(* Logix 5000 AddOnInstructionDefinition export TeNod4TBlocBackupRestore; software revision 28.00 *)

ADD_ON_INSTRUCTION TeNod4TBlocBackupRestore   (* revision 1.1, vendor Scaime *)
VAR_IN_OUT
   Datas : TeNod4TDatas; {required}
END_VAR
VAR_INPUT
   Backup : BOOL; {visible}
   Restore : BOOL; {visible}
END_VAR
VAR_OUTPUT
   InProgress : BOOL; {visible}
   Done : BOOL; {visible}
   Error : BOOL; {visible}
END_VAR
VAR
   IntBackup : BOOL; {access None}
   IntRestore1 : BOOL; {access None}
   IntRestore2 : BOOL; {access None}
   IntRestore3 : BOOL; {access None}
   IntRestore4 : BOOL; {access None}
END_VAR

ROUTINE Logic   (* ladder *)
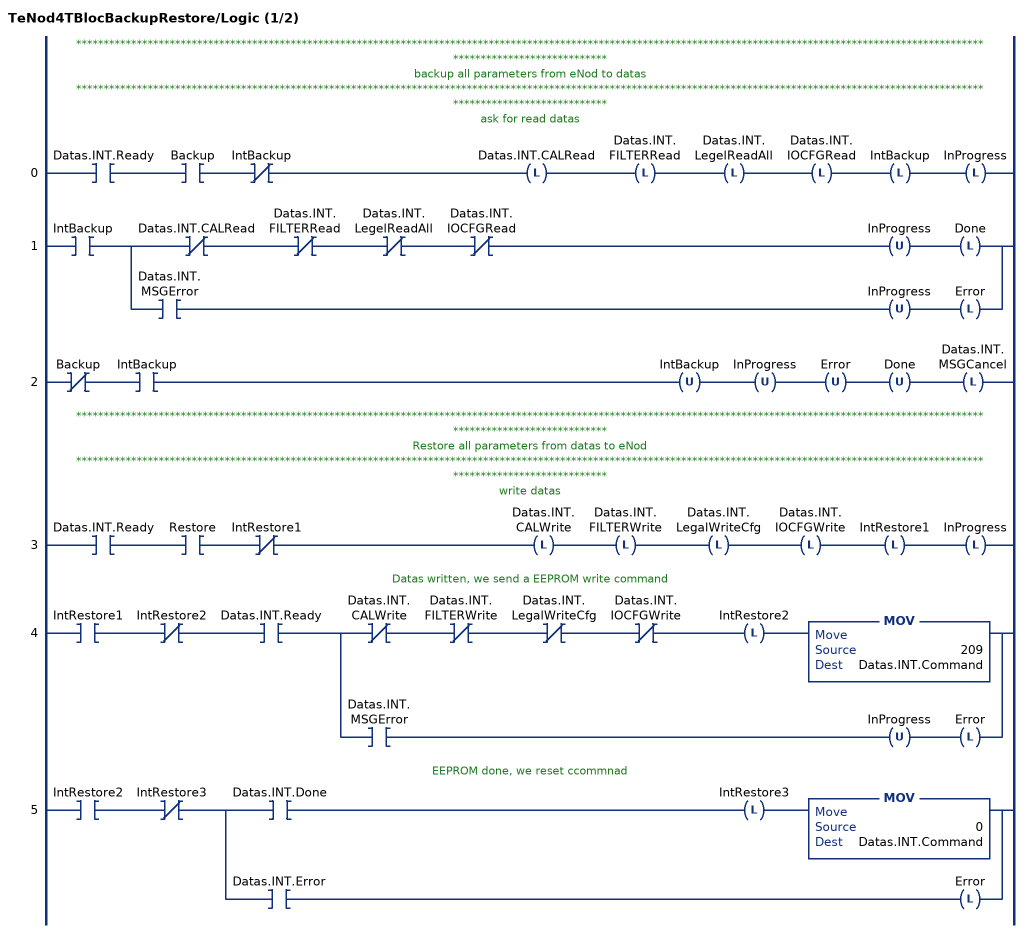
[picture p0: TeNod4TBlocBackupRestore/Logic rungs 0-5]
   // *************************************************************************************************************************************************************************************************
   // backup all parameters from eNod to datas
   // *************************************************************************************************************************************************************************************************
   // ask for read datas
   0: XIC(Datas.INT.Ready)XIC(Backup)XIO(IntBackup)OTL(Datas.INT.CALRead)OTL(Datas.INT.FILTERRead)OTL(Datas.INT.LegelReadAll)OTL(Datas.INT.IOCFGRead)OTL(IntBackup)OTL(InProgress);
   1: XIC(IntBackup)[XIO(Datas.INT.CALRead) XIO(Datas.INT.FILTERRead) XIO(Datas.INT.LegelReadAll) XIO(Datas.INT.IOCFGRead) OTU(InProgress) OTL(Done) ,XIC(Datas.INT.MSGError) OTU(InProgress) OTL(Error) ];
   2: XIO(Backup)XIC(IntBackup)OTU(IntBackup)OTU(InProgress)OTU(Error)OTU(Done)OTL(Datas.INT.MSGCancel);
   // *************************************************************************************************************************************************************************************************
   // Restore all parameters from datas to eNod
   // *************************************************************************************************************************************************************************************************
   // write datas
   3: XIC(Datas.INT.Ready)XIC(Restore)XIO(IntRestore1)OTL(Datas.INT.CALWrite)OTL(Datas.INT.FILTERWrite)OTL(Datas.INT.LegalWriteCfg)OTL(Datas.INT.IOCFGWrite)OTL(IntRestore1)OTL(InProgress);
   // Datas written, we send a EEPROM write command
   4: XIC(IntRestore1)XIO(IntRestore2)XIC(Datas.INT.Ready)[XIO(Datas.INT.CALWrite) XIO(Datas.INT.FILTERWrite) XIO(Datas.INT.LegalWriteCfg) XIO(Datas.INT.IOCFGWrite) OTL(IntRestore2) MOV(209,Datas.INT.Command) ,XIC(Datas.INT.MSGError) OTU(InProgress) OTL(Error) ];
   // EEPROM done, we reset ccommnad
   5: XIC(IntRestore2)XIO(IntRestore3)[XIC(Datas.INT.Done) OTL(IntRestore3) MOV(0,Datas.INT.Command) ,XIC(Datas.INT.Error) OTL(Error) ];
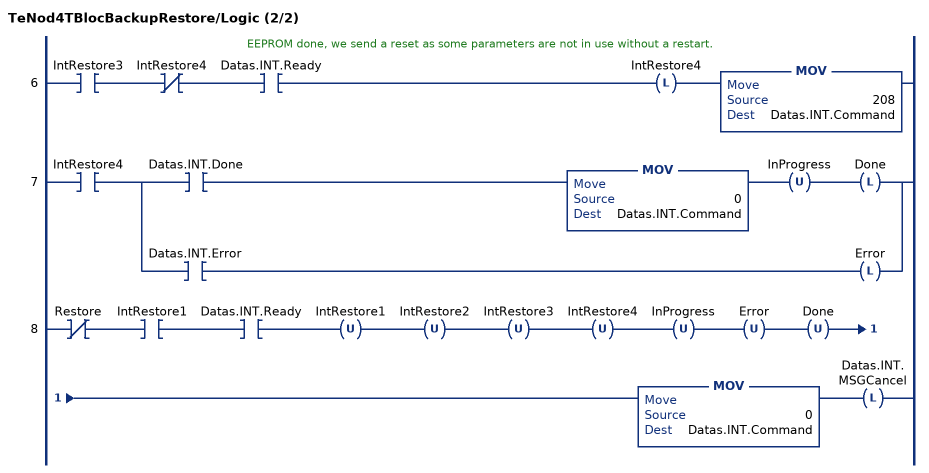
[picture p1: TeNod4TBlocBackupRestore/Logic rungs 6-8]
   // EEPROM done, we send a reset as some parameters are not in use without a restart.
   6: XIC(IntRestore3)XIO(IntRestore4)XIC(Datas.INT.Ready)OTL(IntRestore4)MOV(208,Datas.INT.Command);
   7: XIC(IntRestore4)[XIC(Datas.INT.Done) MOV(0,Datas.INT.Command) OTU(InProgress) OTL(Done) ,XIC(Datas.INT.Error) OTL(Error) ];
   8: XIO(Restore)XIC(IntRestore1)XIC(Datas.INT.Ready)OTU(IntRestore1)OTU(IntRestore2)OTU(IntRestore3)OTU(IntRestore4)OTU(InProgress)OTU(Error)OTU(Done)MOV(0,Datas.INT.Command)OTL(Datas.INT.MSGCancel);
END_ROUTINE
END_ADD_ON_INSTRUCTION
